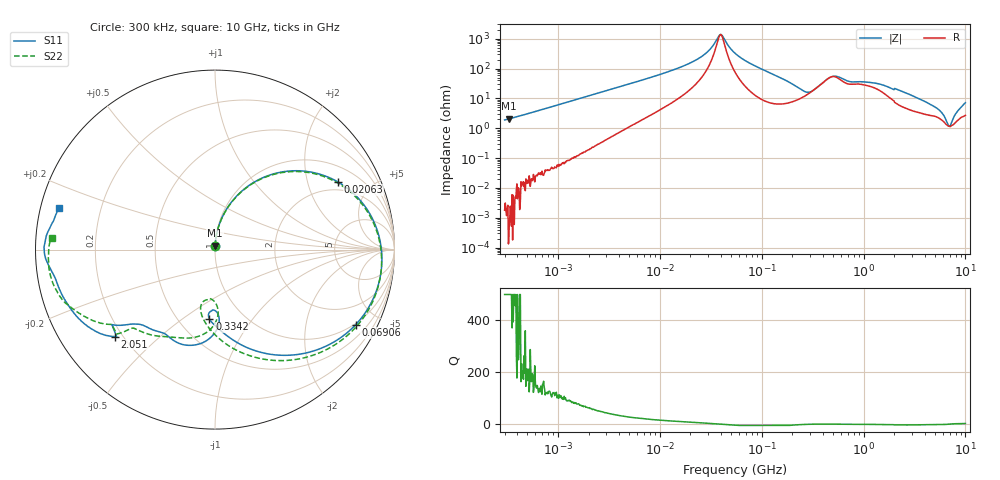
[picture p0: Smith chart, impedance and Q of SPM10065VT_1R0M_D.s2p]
! S-Parameter Data Generated by TDK Corporation
! Copyright(C) 2020 TDK Corporation.
! All Rights Reserved.
! TDK P/N: SPM10065VT-1R0M-D (Inductor)
! Property: L=1uH at 100kHz
! Size(LxWxT): 10.5x10x6.5mm
! Model Type: s2p (Touchstone File Format Version 1.0)
! Frequency: DC=Yes Start=0.3MHz Stop=10000MHz 802points Log-sweep
! Model Generated on Apr. 23, 2020
! Port Assignments:
!  1 ---@@@--- 2
! Applicable Conditions:
!  Temperature = 25 degC
!  DC Bias Current = 0 A
!  Small Signal Operation
! Terms and conditions regarding TDK Simulation Models
! (1)This simulation model is being provided solely for informational purposes. Please refer to the specifications of the products in terms of detailed characteristics of such products.
! (2)In no event shall TDK Corporation of any of its subsidiaries be liable for any loss or damage arising, directly or indirectly,
!  From any information contained in this simulation model, including, but not limited to loss or damages arising from any inaccuracies, omissions or errors in connection with such information.
! (3)Any and all copyrights on this simulation model are owned by TDK Corporation.
!  Duplication or redistribution of this simulation model without prior written permission from TDK Corporation is prohibited.
! (4)This simulation model is subject to any modification or change without any prior notice.
! (5)Neither TDK Corporation nor any of its subsidiaries shall make any warranty, express or implied,
!  Including but not limited to the correctness, implied warranties of merchantability and fitness for a particular purpose with respect to this simulation models.
! (6)The use of this simulation model shall be deemed to have consented to the terms and conditions hereof.
# Hz S MA R 50
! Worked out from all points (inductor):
!   801 points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, 300 kHz to 10 GHz, reference 50 ohm
!   read as 1/Y11, port 2 shorted: L = 981 nH near 318.3 kHz
!   highest Q = 1.66e+03 at 332.1 kHz (marker M1), where L = 993 nH
!   self-resonance near 39.61 MHz
!   S11 on the Smith chart (normalised r, x): 300 kHz: 1.00, +0.04; 20.63 MHz: 1.61, +3.13; 69.06 MHz: 0.95, -3.77; 334.2 MHz: 0.70, -0.64; 2.051 GHz: 0.17, -0.36; 10 GHz: 0.05, +0.13
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300000  0.01949 91.1  0.999 -1.0  0.9994 -1.1  0.01943 90.3
332090  0.02123 90.3  0.9992 -1.1  0.9993 -1.2  0.02111 90.1
1713600  0.1001 83.2  0.9937 -6.0  0.9934 -6.0  0.1002 83.1
4796912  0.2694 71.6  0.9537 -16.4  0.9531 -16.4  0.2694 71.4
9671944  0.4906 55.6  0.8408 -30.9  0.8406 -30.9  0.4907 55.3
2.063197e7  0.7821 28.8  0.5309 -54.3  0.5307 -54.3  0.7821 28.0
3.162388e7  0.8979 10.2  0.2629 -65.3  0.2628 -65.3  0.898 8.9
4.442572e7  0.9332 -5.9  0.06674 -13.3  0.06671 -13.3  0.9332 -7.7
5.477226e7  0.9247 -16.3  0.1604 49.2  0.1604 49.2  0.9248 -18.5
6.905691e7  0.8882 -28.1  0.3188 49.4  0.3187 49.4  0.8879 -30.9
1.080141e8  0.7497 -51.0  0.585 30.6  0.5848 30.6  0.7477 -55.4
1.69821e8  0.5742 -71.9  0.7451 6.9  0.7448 6.9  0.5654 -78.9
3.126428e8  0.4049 -92.6  0.7524 -28.4  0.7521 -28.4  0.3518 -103.0
3.342219e8  0.3886 -94.6  0.734 -32.4  0.7337 -32.4  0.3271 -104.1
4.20949e8  0.3393 -90.1  0.6703 -45.1  0.67 -45.1  0.2794 -93.1
5.497689e8  0.473 -91.0  0.5431 -61.1  0.5429 -61.1  0.3992 -89.2
7.400828e8  0.5557 -114.9  0.4505 -68.5  0.4504 -68.5  0.5202 -108.6
1.10164e9  0.5712 -129.9  0.3839 -94.6  0.3838 -94.6  0.5915 -126.4
1.767019e9  0.6585 -140.4  0.248 -141.9  0.2479 -141.9  0.669 -137.5
2.051294e9  0.7378 -138.9  0.1868 -160.1  0.1867 -160.0  0.7162 -144.4
5.099159e9  0.9052 -170.1  0.01784 164.1  0.01782 164.1  0.9122 -165.5
1e10  0.8996 165.1  0.01789 133.5  0.01782 133.8  0.9112 176.0
